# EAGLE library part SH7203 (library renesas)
Renesas 32-Bit RISC Microcomputer SuperH (TM) RISC engine Family SH7200 Series Auto generated by make-symbol-device-package-bsdl.ulp Rev. 27 Source: rej09b0313_sh7203hm.pdf; sh7203_pin_arrangement.pdf
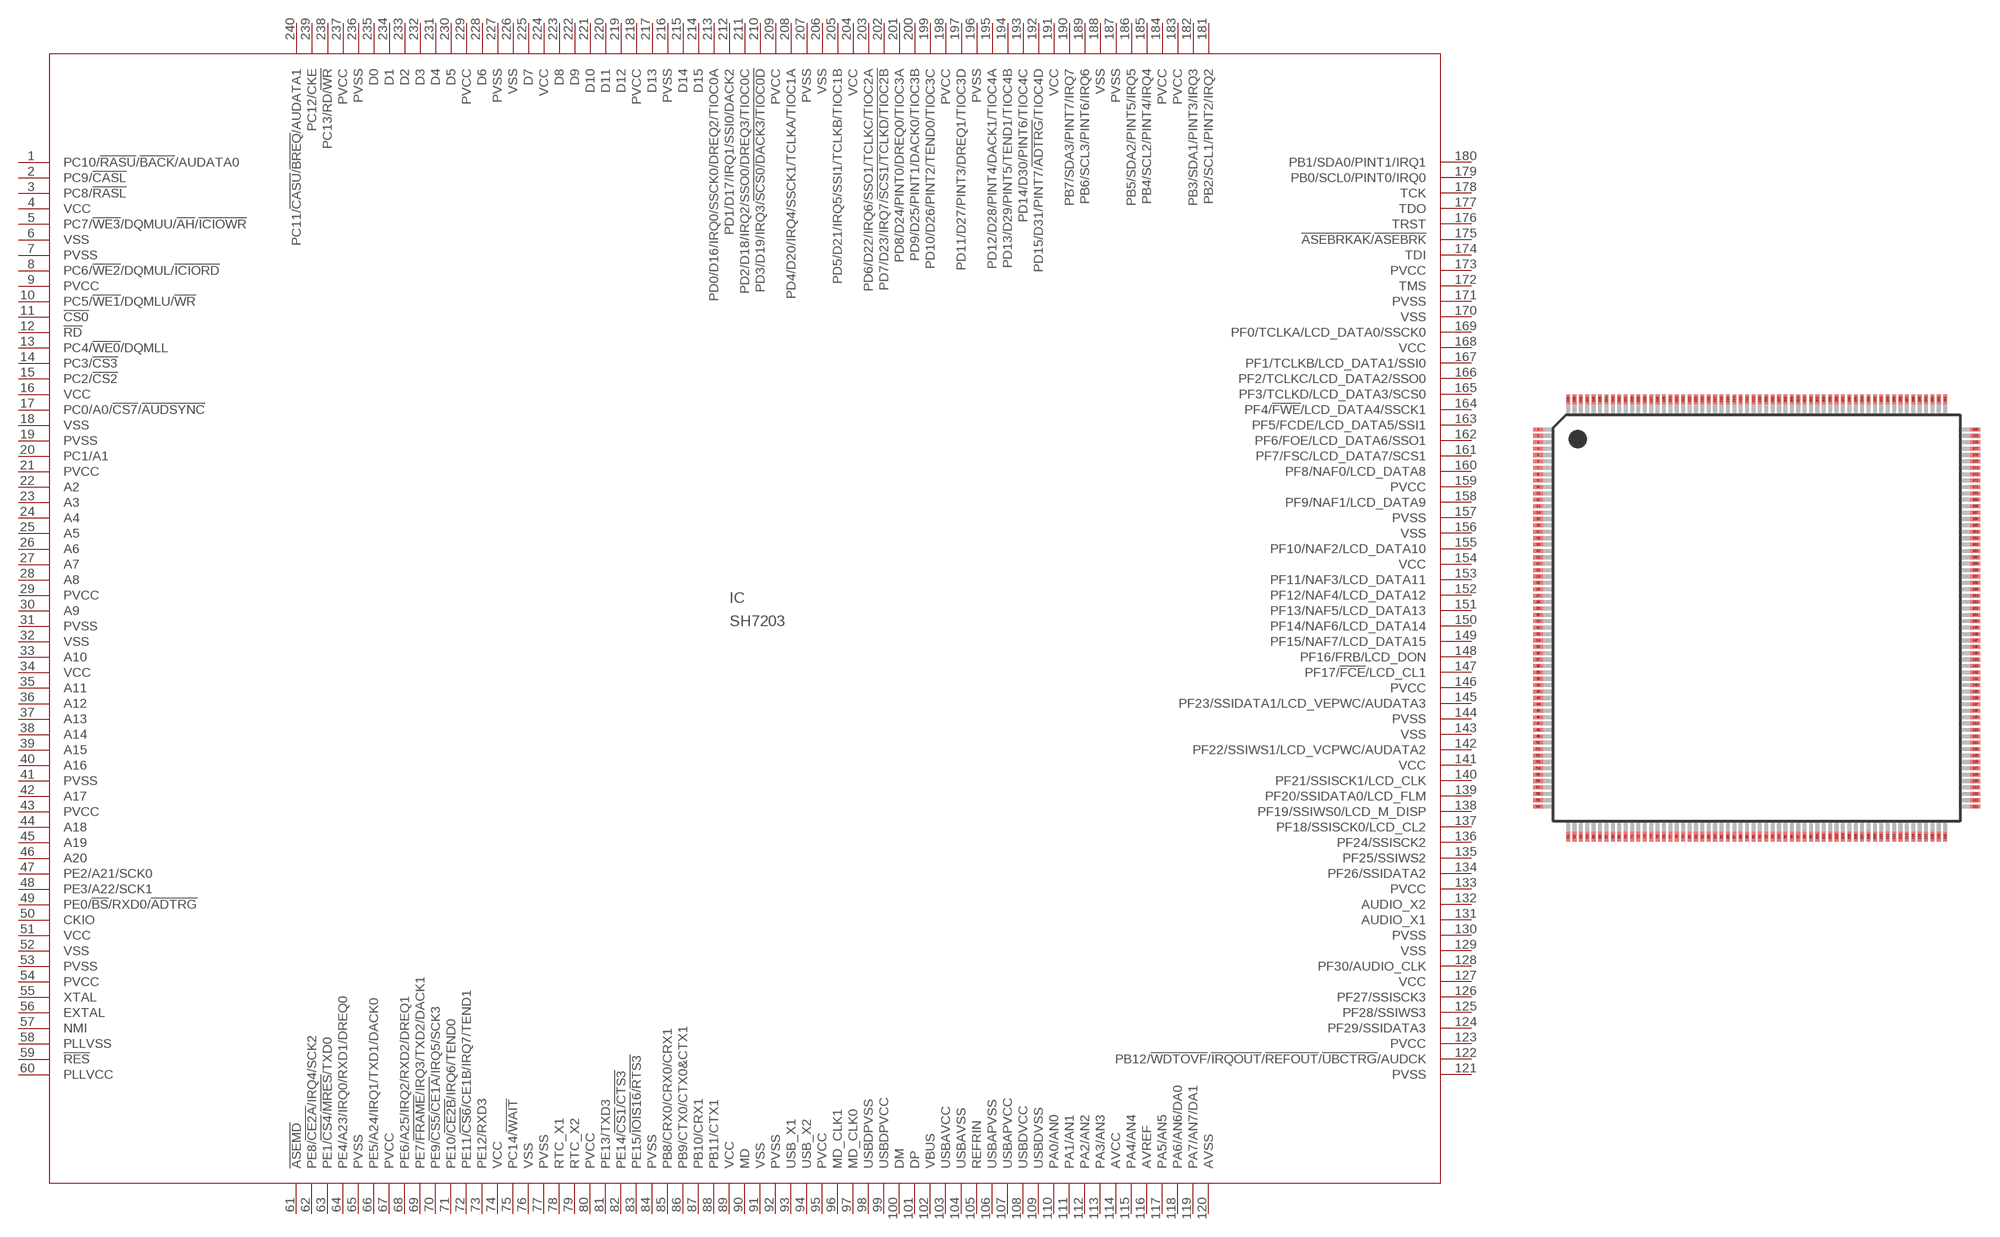
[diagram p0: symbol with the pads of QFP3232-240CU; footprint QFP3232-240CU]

Designator prefix IC

## SH7203 (MPN: DS72030W200FPV; OC_FARNELL: 1677756; OC_NEWARK: 40P2895)  [QFP3232-240CU]
1  PC10/!RASU!/!BACK!/AUDATA0
2  PC9/!CASL
3  PC8/!RASL
4  VCC  pwr
5  PC7/!WE3!/DQMUU/!AH!/!ICIOWR
6  VSS  pwr
7  PVSS  pwr
8  PC6/!WE2!/DQMUL/!ICIORD
9  PVCC  pwr
10  PC5/!WE1!/DQMLU/!WR
11  !CS0  out
12  !RD  out
13  PC4/!WE0!/DQMLL
14  PC3/!CS3
15  PC2/!CS2
16  VCC  pwr
17  PC0/A0/!CS7!/!AUDSYNC
18  VSS  pwr
19  PVSS  pwr
20  PC1/A1
21  PVCC  pwr
22  A2  out
23  A3  out
24  A4  out
25  A5  out
26  A6  out
27  A7  out
28  A8  out
29  PVCC  pwr
30  A9  out
31  PVSS  pwr
32  VSS  pwr
33  A10  out
34  VCC  pwr
35  A11  out
36  A12  out
37  A13  out
38  A14  out
39  A15  out
40  A16  out
41  PVSS  pwr
42  A17  out
43  PVCC  pwr
44  A18  out
45  A19  out
46  A20  out
47  PE2/A21/SCK0
48  PE3/A22/SCK1
49  PE0/!BS!/RXD0/!ADTRG
50  CKIO
51  VCC  pwr
52  VSS  pwr
53  PVSS  pwr
54  PVCC  pwr
55  XTAL  out
56  EXTAL  in
57  NMI  in
58  PLLVSS  pwr
59  !RES  in
60  PLLVCC  pwr
61  !ASEMD  in
62  PE8/!CE2A!/IRQ4/SCK2
63  PE1/!CS4!/!MRES!/TXD0
64  PE4/A23/IRQ0/RXD1/DREQ0
65  PVSS  pwr
66  PE5/A24/IRQ1/TXD1/DACK0
67  PVCC  pwr
68  PE6/A25/IRQ2/RXD2/DREQ1
69  PE7/!FRAME!/IRQ3/TXD2/DACK1
70  PE9/!CS5!/!CE1A!/IRQ5/SCK3
71  PE10/!CE2B!/IRQ6/TEND0
72  PE11/!CS6!/CE1B/IRQ7/TEND1
73  PE12/RXD3
74  VCC  pwr
75  PC14/!WAIT
76  VSS  pwr
77  PVSS  pwr
78  RTC_X1  in
79  RTC_X2  out
80  PVCC  pwr
81  PE13/TXD3
82  PE14/!CS1!/!CTS3
83  PE15/!IOIS16!/!RTS3
84  PVSS  pwr
85  PB8/CRX0/CRX0/CRX1
86  PB9/CTX0/CTX0&CTX1
87  PB10/CRX1
88  PB11/CTX1
89  VCC  pwr
90  MD  in
91  VSS  pwr
92  PVSS  pwr
93  USB_X1  in
94  USB_X2  out
95  PVCC  pwr
96  MD_CLK1  in
97  MD_CLK0  in
98  USBDPVSS  pwr
99  USBDPVCC  pwr
100  DM
101  DP
102  VBUS  in
103  USBAVCC  pwr
104  USBAVSS  pwr
105  REFRIN  in
106  USBAPVSS  pwr
107  USBAPVCC  pwr
108  USBDVCC  pwr
109  USBDVSS  pwr
110  PA0/AN0  in
111  PA1/AN1  in
112  PA2/AN2  in
113  PA3/AN3  in
114  AVCC  pwr
115  PA4/AN4  in
116  AVREF  in
117  PA5/AN5  in
118  PA6/AN6/DA0
119  PA7/AN7/DA1
120  AVSS  pwr
121  PVSS  pwr
122  PB12/!WDTOVF!/!IRQOUT!/!REFOUT!/!UBCTRG!/AUDCK  out
123  PVCC  pwr
124  PF29/SSIDATA3
125  PF28/SSIWS3
126  PF27/SSISCK3
127  VCC  pwr
128  PF30/AUDIO_CLK
129  VSS  pwr
130  PVSS  pwr
131  AUDIO_X1  in
132  AUDIO_X2  out
133  PVCC  pwr
134  PF26/SSIDATA2
135  PF25/SSIWS2
136  PF24/SSISCK2
137  PF18/SSISCK0/LCD_CL2
138  PF19/SSIWS0/LCD_M_DISP
139  PF20/SSIDATA0/LCD_FLM
140  PF21/SSISCK1/LCD_CLK
141  VCC  pwr
142  PF22/SSIWS1/LCD_VCPWC/AUDATA2
143  VSS  pwr
144  PVSS  pwr
145  PF23/SSIDATA1/LCD_VEPWC/AUDATA3
146  PVCC  pwr
147  PF17/!FCE!/LCD_CL1
148  PF16/FRB/LCD_DON
149  PF15/NAF7/LCD_DATA15
150  PF14/NAF6/LCD_DATA14
151  PF13/NAF5/LCD_DATA13
152  PF12/NAF4/LCD_DATA12
153  PF11/NAF3/LCD_DATA11
154  VCC  pwr
155  PF10/NAF2/LCD_DATA10
156  VSS  pwr
157  PVSS  pwr
158  PF9/NAF1/LCD_DATA9
159  PVCC  pwr
160  PF8/NAF0/LCD_DATA8
161  PF7/FSC/LCD_DATA7/SCS1
162  PF6/FOE/LCD_DATA6/SSO1
163  PF5/FCDE/LCD_DATA5/SSI1
164  PF4/!FWE!/LCD_DATA4/SSCK1
165  PF3/TCLKD/LCD_DATA3/SCS0
166  PF2/TCLKC/LCD_DATA2/SSO0
167  PF1/TCLKB/LCD_DATA1/SSI0
168  VCC  pwr
169  PF0/TCLKA/LCD_DATA0/SSCK0
170  VSS  pwr
171  PVSS  pwr
172  TMS  in
173  PVCC  pwr
174  TDI  in
175  !ASEBRKAK!/!ASEBRK
176  TRST  in
177  TDO  out
178  TCK  in
179  PB0/SCL0/PINT0/IRQ0
180  PB1/SDA0/PINT1/IRQ1
181  PB2/SCL1/PINT2/IRQ2
182  PB3/SDA1/PINT3/IRQ3
183  PVCC  pwr
184  PVCC  pwr
185  PB4/SCL2/PINT4/IRQ4
186  PB5/SDA2/PINT5/IRQ5
187  PVSS  pwr
188  VSS  pwr
189  PB6/SCL3/PINT6/IRQ6
190  PB7/SDA3/PINT7/IRQ7
191  VCC  pwr
192  PD15/D31/PINT7/!ADTRG!/TIOC4D
193  PD14/D30/PINT6/TIOC4C
194  PD13/D29/PINT5/TEND1/TIOC4B
195  PD12/D28/PINT4/DACK1/TIOC4A
196  PVSS  pwr
197  PD11/D27/PINT3/DREQ1/TIOC3D
198  PVCC  pwr
199  PD10/D26/PINT2/TEND0/TIOC3C
200  PD9/D25/PINT1/DACK0/TIOC3B
201  PD8/D24/PINT0/DREQ0/TIOC3A
202  PD7/D23/IRQ7/!SCS1/TCLKD/TIOC2B
203  PD6/D22/IRQ6/SSO1/TCLKC/TIOC2A
204  VCC  pwr
205  PD5/D21/IRQ5/SSI1/TCLKB/TIOC1B
206  VSS  pwr
207  PVSS  pwr
208  PD4/D20/IRQ4/SSCK1/TCLKA/TIOC1A
209  PVCC  pwr
210  PD3/D19/IRQ3/!SCS0/DACK3/TIOC0D
211  PD2/D18/IRQ2/SSO0/DREQ3/TIOC0C
212  PD1/D17/IRQ1/SSI0/DACK2  out
213  PD0/D16/IRQ0/SSCK0/DREQ2/TIOC0A
214  D15
215  D14
216  PVSS  pwr
217  D13
218  PVCC  pwr
219  D12
220  D11
221  D10
222  D9
223  D8
224  VCC  pwr
225  D7
226  VSS  pwr
227  PVSS  pwr
228  D6
229  PVCC  pwr
230  D5
231  D4
232  D3
233  D2
234  D1
235  D0
236  PVSS  pwr
237  PVCC  pwr
238  PC13/RD/!WR
239  PC12/CKE
240  PC11/!CASU!/!BREQ!/AUDATA1

## Footprint QFP3232-240CU (pad centres in mm)
JEITA Package Code P-QFP240-32x32-0.50 Source: http://america.renesas.com .. prqp0240ka_a.pdf
smd 0.8 x 0.3: 1 -17.1,14.75; 2 -17.1,14.25; 3 -17.1,13.75; 4 -17.1,13.25; 5 -17.1,12.75; 6 -17.1,12.25; 7 -17.1,11.75; 8 -17.1,11.25; 9 -17.1,10.75; 10 -17.1,10.25; 11 -17.1,9.75; 12 -17.1,9.25; 13 -17.1,8.75; 14 -17.1,8.25; 15 -17.1,7.75; 16 -17.1,7.25; 17 -17.1,6.75; 18 -17.1,6.25; 19 -17.1,5.75; 20 -17.1,5.25; 21 -17.1,4.75; 22 -17.1,4.25; 23 -17.1,3.75; 24 -17.1,3.25; 25 -17.1,2.75; 26 -17.1,2.25; 27 -17.1,1.75; 28 -17.1,1.25; 29 -17.1,0.75; 30 -17.1,0.25; 31 -17.1,-0.25; 32 -17.1,-0.75; 33 -17.1,-1.25; 34 -17.1,-1.75; 35 -17.1,-2.25; 36 -17.1,-2.75; 37 -17.1,-3.25; 38 -17.1,-3.75; 39 -17.1,-4.25; 40 -17.1,-4.75; 41 -17.1,-5.25; 42 -17.1,-5.75; 43 -17.1,-6.25; 44 -17.1,-6.75; 45 -17.1,-7.25; 46 -17.1,-7.75; 47 -17.1,-8.25; 48 -17.1,-8.75; 49 -17.1,-9.25; 50 -17.1,-9.75; 51 -17.1,-10.25; 52 -17.1,-10.75; 53 -17.1,-11.25; 54 -17.1,-11.75; 55 -17.1,-12.25; 56 -17.1,-12.75; 57 -17.1,-13.25; 58 -17.1,-13.75; 59 -17.1,-14.25; 60 -17.1,-14.75; 121 17.1,-14.75; 122 17.1,-14.25; 123 17.1,-13.75; 124 17.1,-13.25; 125 17.1,-12.75; 126 17.1,-12.25; 127 17.1,-11.75; 128 17.1,-11.25; 129 17.1,-10.75; 130 17.1,-10.25; 131 17.1,-9.75; 132 17.1,-9.25; 133 17.1,-8.75; 134 17.1,-8.25; 135 17.1,-7.75; 136 17.1,-7.25; 137 17.1,-6.75; 138 17.1,-6.25; 139 17.1,-5.75; 140 17.1,-5.25; 141 17.1,-4.75; 142 17.1,-4.25; 143 17.1,-3.75; 144 17.1,-3.25; 145 17.1,-2.75; 146 17.1,-2.25; 147 17.1,-1.75; 148 17.1,-1.25; 149 17.1,-0.75; 150 17.1,-0.25; 151 17.1,0.25; 152 17.1,0.75; 153 17.1,1.25; 154 17.1,1.75; 155 17.1,2.25; 156 17.1,2.75; 157 17.1,3.25; 158 17.1,3.75; 159 17.1,4.25; 160 17.1,4.75; 161 17.1,5.25; 162 17.1,5.75; 163 17.1,6.25; 164 17.1,6.75; 165 17.1,7.25; 166 17.1,7.75; 167 17.1,8.25; 168 17.1,8.75; 169 17.1,9.25; 170 17.1,9.75; 171 17.1,10.25; 172 17.1,10.75; 173 17.1,11.25; 174 17.1,11.75; 175 17.1,12.25; 176 17.1,12.75; 177 17.1,13.25; 178 17.1,13.75; 179 17.1,14.25; 180 17.1,14.75
smd 0.3 x 0.8: 61 -14.75,-17.1; 62 -14.25,-17.1; 63 -13.75,-17.1; 64 -13.25,-17.1; 65 -12.75,-17.1; 66 -12.25,-17.1; 67 -11.75,-17.1; 68 -11.25,-17.1; 69 -10.75,-17.1; 70 -10.25,-17.1; 71 -9.75,-17.1; 72 -9.25,-17.1; 73 -8.75,-17.1; 74 -8.25,-17.1; 75 -7.75,-17.1; 76 -7.25,-17.1; 77 -6.75,-17.1; 78 -6.25,-17.1; 79 -5.75,-17.1; 80 -5.25,-17.1; 81 -4.75,-17.1; 82 -4.25,-17.1; 83 -3.75,-17.1; 84 -3.25,-17.1; 85 -2.75,-17.1; 86 -2.25,-17.1; 87 -1.75,-17.1; 88 -1.25,-17.1; 89 -0.75,-17.1; 90 -0.25,-17.1; 91 0.25,-17.1; 92 0.75,-17.1; 93 1.25,-17.1; 94 1.75,-17.1; 95 2.25,-17.1; 96 2.75,-17.1; 97 3.25,-17.1; 98 3.75,-17.1; 99 4.25,-17.1; 100 4.75,-17.1; 101 5.25,-17.1; 102 5.75,-17.1; 103 6.25,-17.1; 104 6.75,-17.1; 105 7.25,-17.1; 106 7.75,-17.1; 107 8.25,-17.1; 108 8.75,-17.1; 109 9.25,-17.1; 110 9.75,-17.1; 111 10.25,-17.1; 112 10.75,-17.1; 113 11.25,-17.1; 114 11.75,-17.1; 115 12.25,-17.1; 116 12.75,-17.1; 117 13.25,-17.1; 118 13.75,-17.1; 119 14.25,-17.1; 120 14.75,-17.1; 181 14.75,17.1; 182 14.25,17.1; 183 13.75,17.1; 184 13.25,17.1; 185 12.75,17.1; 186 12.25,17.1; 187 11.75,17.1; 188 11.25,17.1; 189 10.75,17.1; 190 10.25,17.1; 191 9.75,17.1; 192 9.25,17.1; 193 8.75,17.1; 194 8.25,17.1; 195 7.75,17.1; 196 7.25,17.1; 197 6.75,17.1; 198 6.25,17.1; 199 5.75,17.1; 200 5.25,17.1; 201 4.75,17.1; 202 4.25,17.1; 203 3.75,17.1; 204 3.25,17.1; 205 2.75,17.1; 206 2.25,17.1; 207 1.75,17.1; 208 1.25,17.1; 209 0.75,17.1; 210 0.25,17.1; 211 -0.25,17.1; 212 -0.75,17.1; 213 -1.25,17.1; 214 -1.75,17.1; 215 -2.25,17.1; 216 -2.75,17.1; 217 -3.25,17.1; 218 -3.75,17.1; 219 -4.25,17.1; 220 -4.75,17.1; 221 -5.25,17.1; 222 -5.75,17.1; 223 -6.25,17.1; 224 -6.75,17.1; 225 -7.25,17.1; 226 -7.75,17.1; 227 -8.25,17.1; 228 -8.75,17.1; 229 -9.25,17.1; 230 -9.75,17.1; 231 -10.25,17.1; 232 -10.75,17.1; 233 -11.25,17.1; 234 -11.75,17.1; 235 -12.25,17.1; 236 -12.75,17.1; 237 -13.25,17.1; 238 -13.75,17.1; 239 -14.25,17.1; 240 -14.75,17.1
